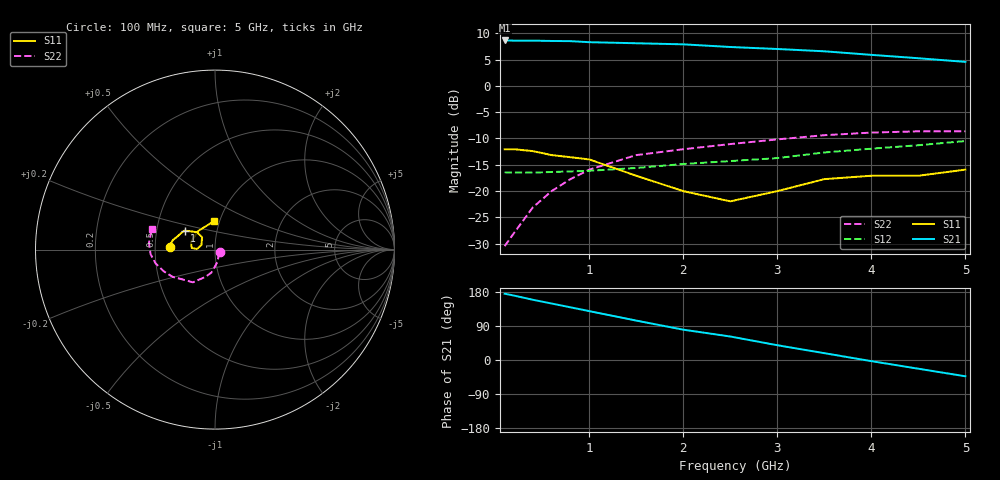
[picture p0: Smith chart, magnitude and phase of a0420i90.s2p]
!  MSA-0420 S AND NOISE PARAMETERS
!  Id=90mA  LAST UPDATED 07-22-92
# ghz s ma r 50
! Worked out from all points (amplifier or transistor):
!   14 points, 100 MHz to 5 GHz, reference 50 ohm
!   highest |S21| = 8.6 dB at 100 MHz (marker M1)
!   |S21| within 3 dB of that: start of sweep to 4.205 GHz
!   unconditionally stable (mu >= 1): start of sweep to end of sweep
!   at 400 MHz: K = 1.36, MAG = 9.0 dB, |S12| = -16.5 dB
!   at 2 GHz: K = 1.25, MAG = 8.3 dB, |S12| = -14.8 dB
!   at 5 GHz: K = 1.03, MAG = 6.5 dB, |S12| = -10.5 dB
!   lowest NFmin = 6.20 dB at 100 MHz
!   S11 on the Smith chart (normalised r, x): 100 MHz: 0.60, +0.02; 1 GHz: 0.70, +0.15; 5 GHz: 0.94, +0.31
0.1  0.25 177.0  2.7 175.0  0.151 1.0  0.03 -30.0
0.2  0.25 173.0  2.69 170.0  0.15 1.0  0.04 -59.0
0.4  0.24 167.0  2.69 159.0  0.15 -1.0  0.07 -79.0
0.6  0.22 160.0  2.67 149.0  0.152 -2.0  0.1 -92.0
0.8  0.21 154.0  2.66 139.0  0.154 -2.0  0.13 -99.0
1  0.2 148.0  2.6 129.0  0.156 -3.0  0.16 -109.0
1.5  0.14 136.0  2.54 104.0  0.166 -4.0  0.22 -124.0
2  0.1 136.0  2.48 80.0  0.181 -6.0  0.25 -139.0
2.5  0.08 161.0  2.34 62.0  0.193 -5.0  0.28 -147.0
3  0.1 178.0  2.24 39.0  0.206 -11.0  0.31 -157.0
3.5  0.13 176.0  2.13 18.0  0.233 -18.0  0.34 -167.0
4  0.14 163.0  1.97 -3.0  0.253 -25.0  0.36 -176.0
4.5  0.14 133.0  1.83 -23.0  0.273 -33.0  0.37 174.0
5  0.16 91.0  1.69 -43.0  0.299 -43.0  0.37 162.0
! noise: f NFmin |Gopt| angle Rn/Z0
0.1  6.2  0.11  -179  0.67
0.5  6.2  0.12  -173  0.67
1  6.4  0.14  -165  0.68
2  7.2  0.18  -145  0.7
